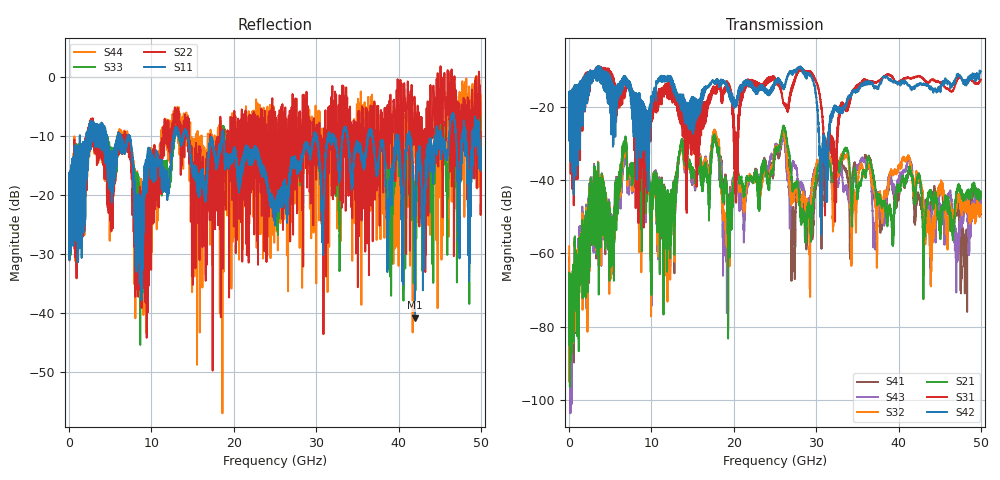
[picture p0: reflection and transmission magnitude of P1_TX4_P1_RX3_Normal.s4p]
!Keysight Technologies,N5225B,MY57041031,A.13.20.10
!Date: Friday, May 31, 2019 11:17:25
!Correction: S11(Full 4 Port(1,2,3,4))
!S12(Full 4 Port(1,2,3,4))
!S13(Full 4 Port(1,2,3,4))
!S14(Full 4 Port(1,2,3,4))
!S21(Full 4 Port(1,2,3,4))
!S22(Full 4 Port(1,2,3,4))
!S23(Full 4 Port(1,2,3,4))
!S24(Full 4 Port(1,2,3,4))
!S31(Full 4 Port(1,2,3,4))
!S32(Full 4 Port(1,2,3,4))
!S33(Full 4 Port(1,2,3,4))
!S34(Full 4 Port(1,2,3,4))
!S41(Full 4 Port(1,2,3,4))
!S42(Full 4 Port(1,2,3,4))
!S43(Full 4 Port(1,2,3,4))
!S44(Full 4 Port(1,2,3,4))
!S4P File: Measurements: <S11,S12,S13,S14>,
!<S21,S22,S23,S24>,
!<S31,S32,S33,S34>,
!<S41,S42,S43,S44>:
# Hz S  dB  R 50.0
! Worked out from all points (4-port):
!   5000 points, 10 MHz to 50 GHz, reference 50 ohm
!   strongest paths, dB at 10 MHz, 12.51 GHz, 25.01 GHz, 37.51 GHz, 50 GHz:
!     S42: -19.6, -14.3, -13.5, -14.8, -10.3
!     S31: -19.6, -17.6, -12.9, -13.1, -12.6
!     S21: -65.6, -45.8, -32.8, -45.6, -43.2
!     S32: -58.1, -47.5, -31.8, -47.4, -47.5
!     S43: -71.8, -49.3, -30.8, -44.0, -45.8
!     S41: -61.0, -47.9, -32.8, -46.8, -48.4
!   lowest |S11| = -40.8 dB at 42 GHz (marker M1), VSWR 1.02, Z = 49.3 + j0.569 ohm
!   |S11| at or under -10 dB: 7.336 GHz to 12.7 GHz (5.362 GHz wide, 53.5 % of centre); 14.41 GHz to 18.57 GHz (4.157 GHz wide, 25.2 % of centre); 18.74 GHz to 29.76 GHz (11.02 GHz wide, 45.4 % of centre)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
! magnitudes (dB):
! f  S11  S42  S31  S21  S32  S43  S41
! 10 MHz  -19.4  -19.6  -19.6  -65.6  -58.1  -71.8  -61.0
! 6.75 GHz  -12.9  -13.5  -16.7  -30.0  -30.9  -32.8  -31.5
! 26.1 GHz  -18.6  -14.3  -19.2  -25.2  -26.9  -28.4  -27.1
! 29.22 GHz  -12.6  -11.1  -10.3  -50.2  -58.4  -45.4  -48.0
! 32.24 GHz  -10.4  -19.8  -35.5  -34.9  -41.0  -39.5  -32.2
! 42 GHz  -40.8  -14.4  -11.9  -45.0  -40.6  -42.1  -50.1
! 50 GHz  -12.0  -10.3  -12.6  -43.2  -47.5  -45.8  -48.4
